FUNCTION_BLOCK FB_LN_IED_LD1_LLN0 EXTENDS FB_AcsiCommonLogicalNodeClass
VAR_INPUT
	NamPlt: FB_DO_IED_LD1_LLN0_NamPlt := (sClass:='LPL', bLinkResult:=THIS^.AddDataToContainer(ipData:=NamPlt));
	Beh: FB_DO_IED_LD1_LLN0_Beh := (sClass:='ENS', bLinkResult:=THIS^.AddDataToContainer(ipData:=Beh));
	Health: FB_DO_IED_LD1_LLN0_Health := (sClass:='ENS', bLinkResult:=THIS^.AddDataToContainer(ipData:=Health));
	Mod_: FB_DO_IED_LD1_LLN0_Mod := (sObjectName:='Mod', sClass:='ENC', bLinkResult:=THIS^.AddDataToContainer(ipData:=Mod_));
END_VAR
VAR
END_VAR

END_FUNCTION_BLOCK
